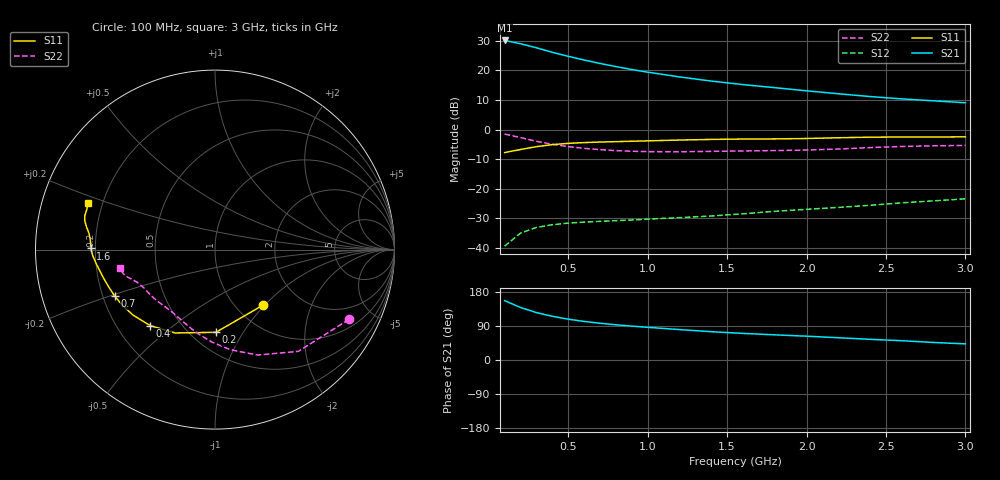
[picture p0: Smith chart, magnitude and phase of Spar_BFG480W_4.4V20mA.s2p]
! Filename: 4_420BFG480.001
! Title: BFG480W
! Bias: Vce=4.4V; Ic=20mA
! Company: NXP Semiconductors NL
! User: Quality&Reliability T&D
! Measure time: 10 Nov 1999 / 12:05:26
#  MHz  S  MA  R 50
! Freq  S11  S21  S12  S22  :
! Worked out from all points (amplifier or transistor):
!   20 points, 100 MHz to 3 GHz, reference 50 ohm
!   highest |S21| = 30.1 dB at 100 MHz (marker M1)
!   |S21| within 3 dB of that: start of sweep to 334.8 MHz
!   unconditionally stable (mu >= 1): 1.349 GHz to end of sweep
!   at 400 MHz: K = 0.41, MSG = 29.1 dB, |S12| = -32.1 dB
!   at 1.2 GHz: K = 0.94, MSG = 23.8 dB, |S12| = -29.7 dB
!   at 3 GHz: K = 1.09, MAG = 14.4 dB, |S12| = -23.4 dB
!   S11 on the Smith chart (normalised r, x): 100 MHz: 1.31, -0.98; 200 MHz: 0.65, -0.77; 400 MHz: 0.34, -0.42; 700 MHz: 0.25, -0.21; 1.6 GHz: 0.18, +0.00; 3 GHz: 0.14, +0.17
100  0.4086 -49.5  31.97 156.7  0.01075 61.0  0.8417 -27.5
200  0.4609 -89.4  28.15 138.6  0.01791 52.4  0.7331 -50.6
300  0.5146 -115.5  24.06 125.1  0.02224 45.7  0.6336 -68.0
400  0.5567 -130.5  20.18 115.3  0.02474 41.7  0.5639 -81.3
500  0.5849 -141.5  17.29 107.8  0.02633 39.8  0.5154 -91.9
600  0.6027 -149.2  14.94 101.8  0.02738 39.1  0.482 -100.2
700  0.6157 -155.1  13.09 97.0  0.02818 39.6  0.4585 -107.0
800  0.6256 -159.8  11.58 92.9  0.02898 40.5  0.4417 -112.8
900  0.6351 -163.6  10.32 89.4  0.02973 42.2  0.4304 -117.9
1000  0.6452 -167.2  9.329 86.2  0.03071 44.0  0.4239 -122.6
1200  0.6652 -172.9  7.749 80.3  0.03259 47.7  0.4221 -130.7
1400  0.6819 -177.1  6.594 74.7  0.03473 51.5  0.4288 -137.1
1600  0.6921 179.5  5.746 70.2  0.03785 55.5  0.4357 -142.0
1800  0.6958 176.0  5.102 66.4  0.04166 59.3  0.4419 -146.8
2000  0.7068 172.8  4.513 62.8  0.04501 62.4  0.4509 -152.1
2200  0.7279 169.8  4.027 58.7  0.04849 64.7  0.4695 -157.1
2400  0.7439 167.4  3.611 54.6  0.05266 66.2  0.4959 -160.9
2600  0.7497 165.3  3.294 50.9  0.05803 67.4  0.5187 -163.4
2800  0.7484 162.7  3.06 46.3  0.06262 67.4  0.531 -165.9
3000  0.7544 159.8  2.837 42.6  0.06771 67.9  0.5402 -169.3
